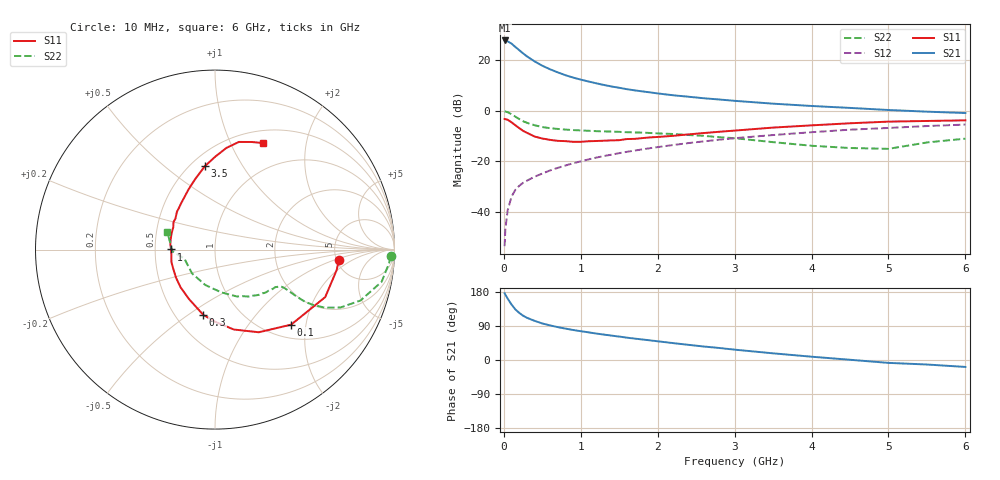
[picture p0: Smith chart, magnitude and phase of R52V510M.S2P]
! SIEMENS Small Signal Semiconductors
! BFR183
! Si NPN RF Bipolar Junction Transistor in SOT23
! VCE = 2.5 V  IC = 10 mA
! Common Emitter S-Parameters:  May  1996
# GHz  S  MA  R  50
!  f  S11  S21  S12  S22
! GHz  MAG  ANG  MAG  ANG  MAG  ANG  MAG  ANG
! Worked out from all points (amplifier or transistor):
!   36 points, 10 MHz to 6 GHz, reference 50 ohm
!   highest |S21| = 27.9 dB at 10 MHz (marker M1)
!   |S21| within 3 dB of that: start of sweep to 166.5 MHz
!   unconditionally stable (mu >= 1): 758.2 MHz to 2.501 GHz
!   at 250 MHz: K = 0.63, MSG = 25.6 dB, |S12| = -28.5 dB
!   at 1.4 GHz: K = 1.06, MAG = 12.1 dB, |S12| = -17.3 dB
!   at 6 GHz: K = 0.90, MSG = 2.3 dB, |S12| = -5.4 dB
!   lowest NFmin = 1.30 dB at 450 MHz
!   S11 on the Smith chart (normalised r, x): 10 MHz: 5.22, -1.18; 100 MHz: 1.27, -1.65; 300 MHz: 0.68, -0.57; 1 GHz: 0.61, +0.00; 3.5 GHz: 0.59, +0.70; 6 GHz: 0.65, +1.33
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0.01  0.692 -4.9  24.88 176.3  0.0021 89.9  0.9786 -2.2
0.02  0.6875 -9.5  24.52 172.4  0.0046 81.0  0.9726 -4.5
0.05  0.6687 -23.3  23.9 161.9  0.0108 79.3  0.9458 -10.9
0.1  0.5956 -44.6  21.53 146.3  0.0201 71.6  0.8587 -19.3
0.15  0.5211 -62.1  18.47 133.5  0.0275 66.5  0.7694 -24.8
0.2  0.4576 -76.7  15.99 124.3  0.0329 63.6  0.6912 -27.9
0.25  0.4034 -89.5  13.81 116.9  0.0377 62.5  0.6268 -29.4
0.3  0.3694 -100.2  12.06 111.4  0.0416 62.2  0.5825 -30.1
0.4  0.3114 -117.7  9.582 103.3  0.0499 62.5  0.5216 -29.9
0.5  0.2843 -132.5  7.859 96.4  0.0576 63.7  0.4797 -29.4
0.6  0.2676 -144.4  6.691 91.3  0.0663 64.6  0.4559 -29.1
0.7  0.2557 -155.8  5.814 86.8  0.0745 64.8  0.4405 -29.0
0.8  0.2524 -164.0  5.11 82.9  0.083 64.8  0.4275 -29.1
1  0.2446 179.8  4.169 76.0  0.1004 65.4  0.4113 -29.8
1.1  0.2513 172.8  3.829 73.0  0.1097 65.5  0.4049 -30.9
1.3  0.2573 160.4  3.27 67.1  0.1278 64.6  0.3935 -32.6
1.6  0.2775 146.4  2.697 58.9  0.1552 62.7  0.3791 -36.5
2.2  0.3214 125.6  2.045 44.6  0.2115 57.9  0.3497 -46.3
3.5  0.4683 96.9  1.394 17.6  0.3335 43.0  0.241 -81.6
4.5  0.5701 83.6  1.148 0.6  0.4257 30.5  0.1845 -133.9
5.5  0.6333 71.2  0.968 -11.9  0.5019 18.6  0.2376 -177.6
6  0.6511 65.8  0.909 -18.3  0.5375 10.8  0.2826 159.8
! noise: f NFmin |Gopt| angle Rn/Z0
0.45  1.3  0.15  45  0.18
0.9  1.4  0.2  125  0.19
1.8  2.1  0.34  -170  0.14
